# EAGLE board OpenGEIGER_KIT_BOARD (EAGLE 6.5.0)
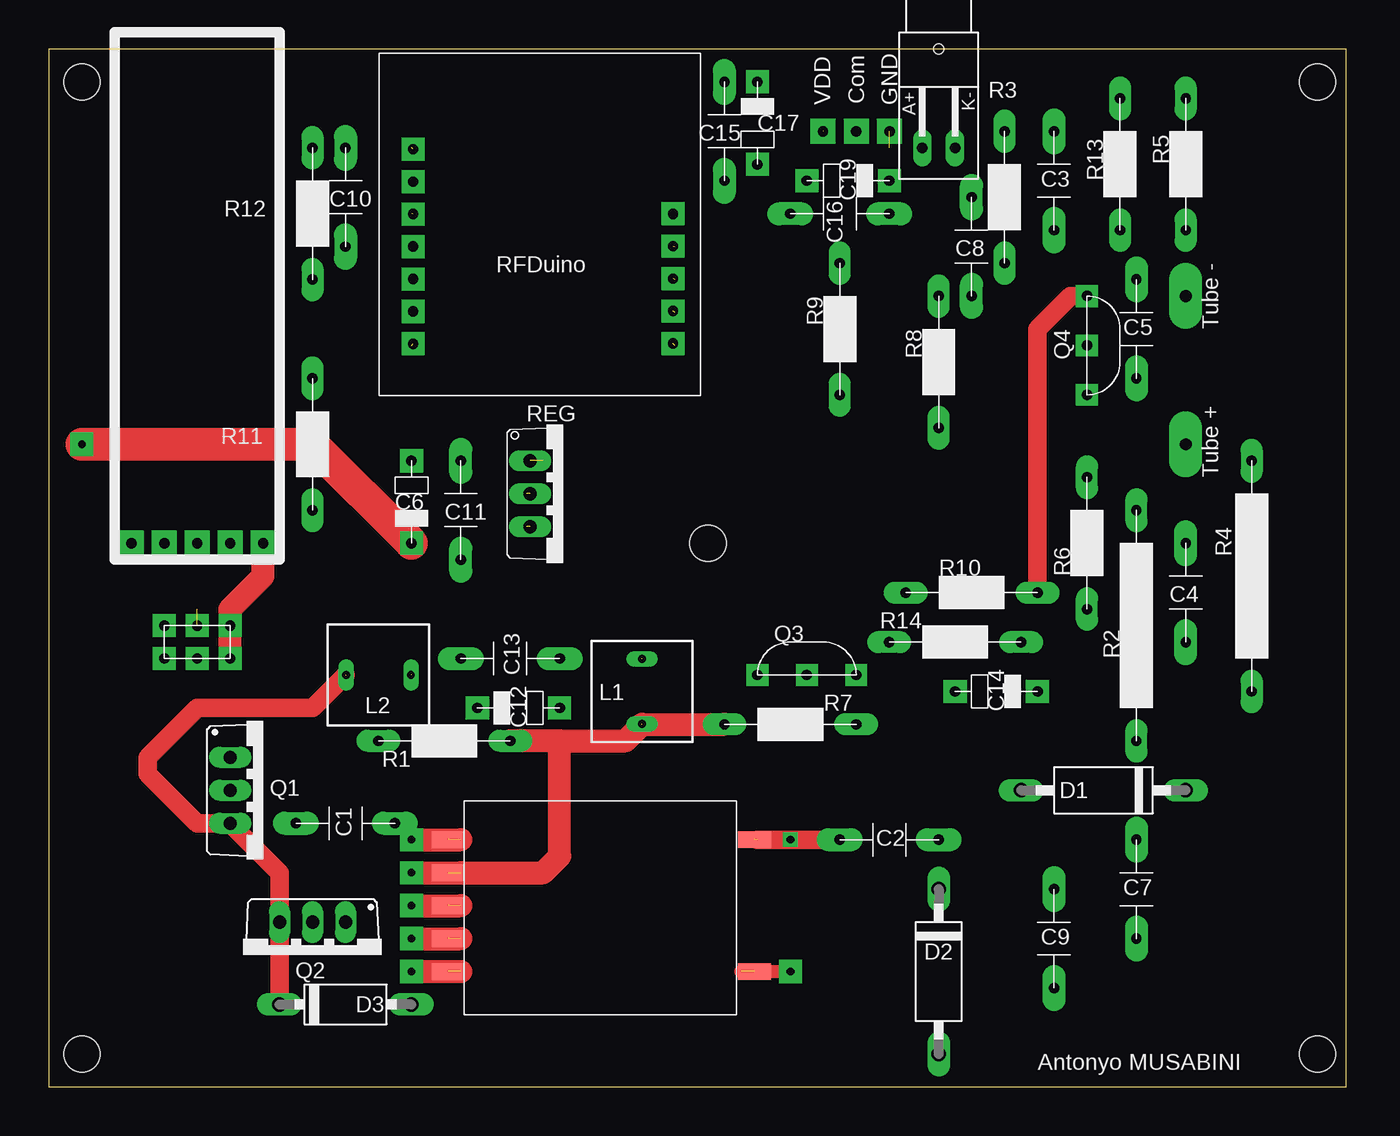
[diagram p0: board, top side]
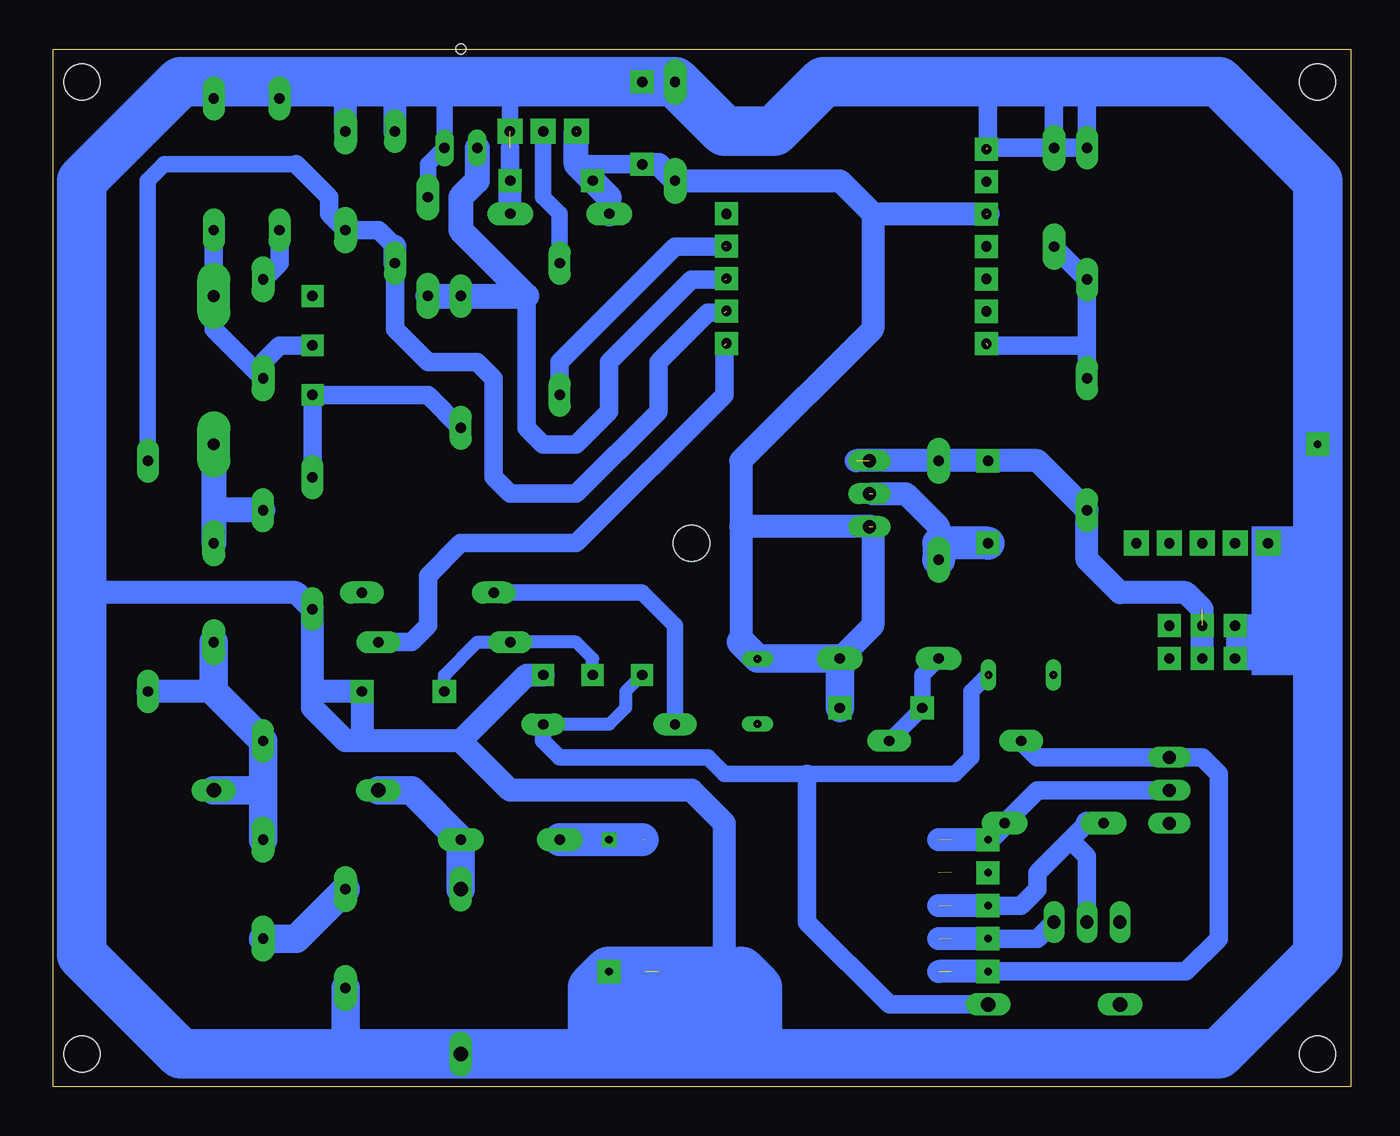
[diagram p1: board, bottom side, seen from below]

Size 100 x 80 mm. Coordinates in mm from the lower left corner, seen from the top.
Outline: 0,0 100,0 100,80 0,80 0,0
Copper layers (1*16): Top 0.035mm / dielectric 1.5mm / Bottom 0.035mm
Design rules "8mils": minimum track width 8mil, minimum drill 20mil, track to track 8mil, track to pad 8mil, pad to pad 8mil, via to via 8mil, smd to smd 8mil, copper to edge 10mil, drill to drill 8mil, minimum pad ring 12mil, minimum via ring 10mil, stop-mask expansion 4mil, vias tented up to drill 25mil, thermal gap 10mil
Holes 2.8 mm at 2.54,77.47 2.54,2.54 97.79,2.54 97.79,77.47 50.8,41.91

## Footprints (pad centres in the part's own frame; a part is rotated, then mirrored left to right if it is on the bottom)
MY_CONDO = drill 0.8 pad 1.778 long: P$1 0,0; P$2 7.62,0
MY_CONDO_CH = drill 0.8 pad 1.778 square: P$1 0,0; P$2 6.35,0
DO15-12 = drill 1.118 long: A 6.35,0; C -6.35,0
P1-10 = drill 1.118 long: A 5.08,0; C -5.08,0
SD8 = drill 0.6 long: 1 -2.5,0; 2 2.5,0
Q62902-B155 = drill 0.813 long: A 7.62,-1.27; K 7.62,1.27 | hole 0.813: 0,0
TO220BV = drill 1.016 long: 1 -2.54,-2.54; 2 0,-2.54; 3 2.54,-2.54
MY_TO92 = drill 0.8 pad 1.676 square: B 3.81,0; C 0,0; E 7.62,0
MY_RESISTANCE = drill 0.8 pad 1.676 long: P$1 0,0; P$2 10.16,0
MY_BIG_R = drill 0.8 pad 1.676 long: P$1 0,0; P$2 17.78,0
TO220V = drill 1.016 long: 1 -2.54,-2.54; 2 0,-2.54; 3 2.54,-2.54
CCFL_TRANSFO = smd 2.54 x 1.27: P$1 -1.238,13.5; P$2 -1.238,10.96; P$3 -1.238,8.42; P$4 -1.238,5.88; P$5 -1.238,3.34; P$6 22.365,3.34; P$10 22.365,13.5
TUBE = drill 0.9 pad 2.54 long: P$1 0,0; P$2 11.43,0
INTERRUPTEUR = drill 0.8 pad 1.778 square: B1 0,-5.08; B2 2.54,-5.08; H1 0,0; H2 2.54,0; M1 0,-2.54; M2 2.54,-2.54
RFDUINO = drill 0.8 pad 1.778 square: +3V 2.606,-12.375; FACTORY 2.606,-17.375; GND 2.606,-7.375; GPIO0/AREF 2.606,-19.875; GPIO1 2.606,-22.375; GPIO2 22.644,-22.35; GPIO3 22.644,-19.85; GPIO4 22.644,-17.35; GPIO5 22.644,-14.85; GPIO6 22.644,-12.35; P2 2.606,-9.875; RESET 2.606,-14.875
CHARGEUR = drill 0.8 pad 1.93 square: P$1 0,0; P$2 0,-2.54; P$3 0,-5.08; P$4 0,-7.62; P$5 0,-10.16
LED_RGB = drill 0.8 pad 1.93 square: COM 0,0; GND 0,2.57; VDD 0,-2.57

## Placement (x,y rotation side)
C1  220n  [MY_CONDO]  19.05,20.32 0 top
C2  47n  [MY_CONDO]  60.96,19.05 0 top
C3  100n  [MY_CONDO]  77.47,73.66 270 top
C4  1n  [MY_CONDO]  87.63,34.29 90 top
C5  10n  [MY_CONDO]  83.82,62.23 270 top
C6  1u  [MY_CONDO_CH]  27.94,48.26 270 top
C7  100n  [MY_CONDO]  83.82,19.05 270 top
C8  100n  [MY_CONDO]  71.12,60.96 90 top
C9  47n  [MY_CONDO]  77.47,15.24 270 top
C10  100n  [MY_CONDO]  22.86,72.39 270 top
C11  100n  [MY_CONDO]  31.75,40.64 90 top
C12  1u  [MY_CONDO_CH]  39.37,29.21 180 top
C13  100n  [MY_CONDO]  31.75,33.02 0 top
C14  1u  [MY_CONDO_CH]  69.85,30.48 0 top
C15  100n  [MY_CONDO]  52.07,77.47 270 top
C16  100n  [MY_CONDO]  64.77,67.31 180 top
C17  1u  [MY_CONDO_CH]  54.61,71.12 90 top
C19  1u  [MY_CONDO_CH]  58.42,69.85 0 top
D1  1N5060GP  [DO15-12]  81.28,22.86 180 top
D2  1N5060GP  [DO15-12]  68.58,8.89 270 top
D3  BA157  [P1-10]  22.86,6.35 0 top
L1  100u  [SD8]  45.72,30.48 90 top
L2  100u  [SD8]  25.4,31.75 180 top
LED1  [Q62902-B155]  68.58,80.01 270 top
Q1  BU505  [TO220BV]  16.51,22.86 270 top
Q2  BU505  [TO220BV]  20.32,10.16 180 top
Q3  BC337  [MY_TO92]  54.61,31.75 0 top
Q4  BC337  [MY_TO92]  80.01,60.96 270 top
R1  330  [MY_RESISTANCE]  25.4,26.67 0 top
R2  4.7M  [MY_BIG_R]  83.82,26.67 90 top
R3  47k  [MY_RESISTANCE]  73.66,73.66 270 top
R4  15M  [MY_BIG_R]  92.71,48.26 270 top
R5  470k  [MY_RESISTANCE]  87.63,76.2 270 top
R6  10k  [MY_RESISTANCE]  80.01,36.83 90 top
R7  1k  [MY_RESISTANCE]  62.23,27.94 180 top
R8  330  [MY_RESISTANCE]  68.58,50.8 90 top
R9  1k  [MY_RESISTANCE]  60.96,53.34 90 top
R10  330  [MY_RESISTANCE]  66.04,38.1 0 top
R11  10k  [MY_RESISTANCE]  20.32,44.45 90 top
R12  33k  [MY_RESISTANCE]  20.32,72.39 270 top
R13  10  [MY_RESISTANCE]  82.55,76.2 270 top
R14  1k  [MY_RESISTANCE]  74.93,34.29 180 top
REG  786TV  [TO220V]  39.62,45.72 270 top
U$1  CCFL_TRANSFO  [CCFL_TRANSFO]  32,5.56 0 top
U$2  TUBE  [TUBE]  87.63,49.53 90 top
U$3  ANTONYO  [ANTONYO]  76.2,1.27 0 top
U$4  INTERRUPTEUR  [INTERRUPTEUR]  13.97,35.56 270 top
U$5  RFDUINO  [RFDUINO]  25.46,79.65 0 top
U$6  CHARGEUR  [CHARGEUR]  6.35,41.91 90 top
U$7  LED_RGB  [LED_RGB]  62.23,73.66 270 top

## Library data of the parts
C1-C17 C19 Q3 Q4 R1-R14 U$1-U$7 = openGeiger
D1-D3 = diode
L1 L2 = inductor-neosid; OC_FARNELL: unknown; OC_NEWARK: unknown
LED1 = led
Q1 Q2 = transistor
REG = linear

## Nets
CHARGEUR+: U$4.H1 U$4.H2 U$6.P$5
COUPS: C8.P$1 LED1.A R8.P$2 U$5.GPIO4
GND: C3.P$1 C6.P$2 C8.P$2 C9.P$2 C10.P$1 C11.P$1 C14.P$2 C15.P$1 C16.P$1 C17.P$2 C19.P$2 D2.A LED1.K Q3.E R3.P$1 R5.P$1 R6.P$1 R12.P$1 R13.P$1 REG.2 U$1.P$6 U$4.B1 U$4.B2 U$5.GND U$6.P$1 U$7.GND
HIGH_V: C4.P$1 C7.P$1 D1.C R2.P$1 R4.P$2
N$1: R9.P$1 U$5.GPIO5
N$2: C7.P$2 C9.P$1
N$3: C2.P$2 D1.A D2.C
N$4: Q1.1 R1.P$1 U$1.P$5
N$5: D3.A L2.1 Q3.C R7.P$1
N$6: C5.P$2 Q4.B R5.P$2 U$2.P$2
N$7: R9.P$2 U$7.COM
N$8: D3.C L2.2 Q1.3 Q2.3
N$9: Q2.1 U$1.P$4
N$10: C10.P$2 R11.P$2 R12.P$2 U$5.GPIO1
N$11: C5.P$1 R13.P$2
N$12: C4.P$2 R2.P$2 U$2.P$1
N$15: Q4.E R6.P$2 R8.P$1
N$17: C1.P$2 Q1.2 U$1.P$1
N$18: C14.P$1 Q3.B R14.P$2
N$19: Q4.C R10.P$2
N$23: C1.P$1 Q2.2 U$1.P$3
N$26: R14.P$1 U$5.GPIO2
N$28: C2.P$1 U$1.P$10
V_SENSE: C3.P$2 R3.P$2 R4.P$1 U$5.GPIO3
VDD_POST_BOBINE: C12.P$2 C13.P$1 L1.1 R1.P$2 R7.P$2 R10.P$1 U$1.P$2
VDD_PRE_REGULATOR: C6.P$1 C11.P$2 R11.P$1 REG.1 U$4.M1 U$4.M2
VDD_PRé_BOBINE: C12.P$1 C13.P$2 C15.P$2 C16.P$2 C17.P$1 C19.P$1 L1.2 REG.3 U$5.+3V U$7.VDD

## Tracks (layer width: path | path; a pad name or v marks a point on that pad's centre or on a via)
CHARGEUR+
  Top 1.778: U$4.H2 U$4.H1 13.97,36.83 16.51,39.37 U$6.P$5
COUPS  (1 unrouted)
  Bottom 1.422: 63.5,60.96 63.5,50.8 62.23,49.53 59.69,49.53 57.15,52.07 57.15,55.88 50.8,62.23 48.26,62.23
  Bottom 1.93: LED1.A 67.31,69.85 68.58,68.58 68.58,66.04 63.5,60.96 R8.P$2 C8.P$1
GND  (via drill 0.6 pad 1.78)  (4 unrouted)
  Top 1.016: 53.34,8.89 v57.15,8.89
  Top 2.54: C6.P$2 20.32,49.53 v2.54,49.53
  Bottom 1.27: R13.P$1 R5.P$1 | C8.P$2 71.12,71.12 LED1.K 69.85,77.47 | 64.77,72.39 64.77,77.47
  Bottom 1.422: C19.P$2 64.77,72.39 | C10.P$1 R12.P$1 20.32,77.47 | C10.P$1 22.86,77.47 | C10.P$1 27.94,72.39 27.94,77.47 | U$4.B2 U$4.B1
  Bottom 1.778: C16.P$1 C19.P$2 | R3.P$1 73.66,77.47 | C3.P$1 77.47,77.47 | R13.P$1 82.55,77.47 | R5.P$1 85.09,77.47 | 77.47,2.54 77.47,3.81 76.2,2.54 D2.A | 46.99,8.89 48.26,8.89 48.26,20.32 50.8,22.86 64.77,22.86 68.58,26.67 | 68.58,26.67 76.2,26.67 | 76.2,26.67 77.47,26.67 80.01,29.21 80.01,30.48 | 80.01,30.48 R6.P$1 81.28,38.1 97.79,38.1 | 68.58,26.67 63.5,31.75 Q3.E | 80.01,30.48 C14.P$2 76.2,26.67 | U$6.P$1 2.54,41.91 | U$4.B1 2.54,35.56 | U$4.B2 2.54,33.02 | 36.83,45.72 34.29,45.72 31.75,43.18 31.75,41.91
  Bottom 2.184: C9.P$2 77.47,3.81
  Bottom 2.54: C11.P$1 31.75,41.91 C6.P$2
  Bottom 3.81: 45.72,2.54 10.16,2.54 2.54,10.16 2.54,33.02 2.54,35.56 2.54,41.91 v2.54,49.53 2.54,69.85 10.16,77.47 20.32,77.47 22.86,77.47 27.94,77.47 40.64,77.47 44.45,73.66 48.26,73.66 C15.P$1 C17.P$2 64.77,77.47 69.85,77.47 73.66,77.47 77.47,77.47 82.55,77.47 85.09,77.47 90.17,77.47 97.79,69.85 97.79,38.1 97.79,10.16 90.17,2.54 77.47,2.54 D2.A 58.42,2.54 | 45.72,2.54 58.42,2.54 | 58.42,2.54 58.42,7.62 v57.15,8.89 48.26,8.89 | 46.99,8.89 45.72,7.62 45.72,2.54
HIGH_V
  Bottom 1.778: 87.63,30.48 R4.P$2
  Bottom 2.184: C4.P$1 87.63,30.48 R2.P$1 83.82,22.86 | 83.82,22.86 C7.P$1 | 83.82,22.86 D1.C
N$1  (1 unrouted)
  Bottom 1.422: R9.P$1 60.96,55.88 52.07,64.77 48.26,64.77
N$2
  Bottom 2.184: C9.P$1 81.28,11.43 C7.P$2
N$3
  Bottom 2.184: D2.C C2.P$2 72.39,22.86 D1.A
N$4  (via drill 0.6 pad 1.78)  (1 unrouted)
  Top 1.778: v27.94,8.89 31.75,8.89
  Bottom 1.422: R1.P$1 24.13,25.4 Q1.1 11.43,25.4 10.16,24.13 10.16,11.43 12.7,8.89 v27.94,8.89
  Bottom 1.778: v27.94,8.89 31.75,8.89
N$5  (1 unrouted)
  Bottom 1.016: Q3.C 55.88,30.48 55.88,29.21 57.15,27.94 R7.P$1
  Bottom 1.27: 27.94,31.75 29.21,30.48 29.21,25.4 30.48,24.13 41.91,24.13 48.26,24.13 49.53,25.4 60.96,25.4 62.23,26.67 R7.P$1
  Bottom 1.422: D3.A 35.56,6.35 41.91,12.7 41.91,24.13
N$6
  Bottom 1.422: R5.P$2 U$2.P$2 87.63,58.42 C5.P$2 83.82,55.88 82.55,57.15 Q4.B
  Bottom 1.93: 87.63,59.69 U$2.P$2
N$7
  Bottom 1.27: R9.P$2 60.96,67.31 62.23,68.58 U$7.COM
N$8  (1 unrouted)
  Top 1.422: D3.C Q2.3 17.78,16.51 Q1.3 11.43,20.32 7.62,24.13 7.62,25.4 11.43,29.21 20.32,29.21 22.86,31.75
N$9  (via drill 0.6 pad 1.78)  (1 unrouted)
  Top 1.778: v27.94,11.43 31.75,11.43
  Bottom 1.422: Q2.1 24.13,11.43 v27.94,11.43
  Bottom 1.778: v27.94,11.43 31.75,11.43
N$10  (1 unrouted)
  Bottom 1.422: C10.P$2 R12.P$2 20.32,57.15 | R11.P$2 20.32,57.15 | 27.94,57.15 20.32,57.15
N$11
  Bottom 1.422: R13.P$2 82.55,63.5 C5.P$1
N$12
  Bottom 1.93: R2.P$2 87.63,44.45 | U$2.P$1 87.63,44.45 | 87.63,44.45 C4.P$2
N$15
  Bottom 1.422: R8.P$1 71.12,53.34 Q4.E R6.P$2
N$17  (via drill 0.6 pad 1.78)  (1 unrouted)
  Top 1.778: v27.94,19.05 31.75,19.05
  Bottom 1.422: Q1.2 24.13,22.86 C1.P$2
  Bottom 1.778: C1.P$2 v27.94,19.05 31.75,19.05
N$18
  Bottom 1.016: Q3.B 58.42,33.02 59.69,34.29 63.5,34.29 R14.P$2 67.31,34.29 69.85,31.75 C14.P$1
N$19
  Top 1.422: Q4.C 78.74,60.96 76.2,58.42 R10.P$2
N$23  (via drill 0.6 pad 1.78)  (1 unrouted)
  Top 1.778: v27.94,13.97 31.75,13.97
  Bottom 1.422: 20.32,13.97 Q2.2 20.32,17.78 21.59,19.05 | 20.32,20.32 21.59,19.05 | 21.59,19.05 24.13,16.51 24.13,15.24 25.4,13.97 v27.94,13.97
  Bottom 1.778: C1.P$1 20.32,20.32 | v27.94,13.97 31.75,13.97
N$26  (1 unrouted)
  Bottom 1.422: 48.26,57.15 48.26,53.34 59.69,41.91 68.58,41.91 71.12,39.37 71.12,35.56 72.39,34.29 R14.P$1
N$28  (via drill 0.6)  (1 unrouted)
  Top 1.422: 54.61,19.05 v57.15,19.05 C2.P$1
  Bottom 2.54: 54.61,19.05 v57.15,19.05 C2.P$1
V_SENSE  (1 unrouted)
  Bottom 1.27: 81.28,71.12 91.44,71.12 92.71,69.85 R4.P$1
  Bottom 1.422: R3.P$2 73.66,58.42 71.12,55.88 67.31,55.88 66.04,54.61 66.04,46.99 64.77,45.72 59.69,45.72 53.34,52.07 53.34,55.88 49.53,59.69 48.26,59.69 | 73.66,64.77 74.93,66.04 C3.P$2 78.74,67.31 78.74,68.58 81.28,71.12
  Bottom 1.778: R3.P$2 73.66,64.77
VDD_POST_BOBINE  (via drill 0.6 pad 1.78)  (2 unrouted)
  Top 1.778: 31.75,16.51 v27.94,16.51 38.1,16.51 39.37,17.78 39.37,26.67 | 39.37,26.67 44.45,26.67 45.72,27.94 R7.P$2 | 39.37,26.67 R1.P$2
  Bottom 1.27: C13.P$1 33.02,31.75 C12.P$2 R1.P$2 | R7.P$2 52.07,35.56 54.61,38.1 R10.P$1
VDD_PRE_REGULATOR  (2 unrouted)
  Bottom 1.778: U$4.M2 11.43,36.83 12.7,38.1 17.78,38.1 20.32,40.64 R11.P$1 24.13,48.26 C6.P$1 C11.P$2 38.1,48.26
VDD_PRé_BOBINE  (4 unrouted)
  Bottom 1.422: C17.P$1 59.69,71.12
  Bottom 1.778: C17.P$1 53.34,71.12 C15.P$2 39.37,69.85 36.83,67.31 | 36.83,67.31 27.94,67.31 | 36.83,67.31 36.83,58.42 46.99,48.26 46.99,43.18 | 46.99,43.18 46.99,34.29 | 46.99,43.18 36.83,43.18 36.83,35.56 C13.P$2
  Bottom 1.93: C16.P$2 57.15,68.58 C19.P$1 59.69,71.12 59.69,73.66
  Bottom 2.184: C12.P$1 C13.P$2 45.72,33.02 46.99,34.29
(copper drawn outside any net)
  shapes: Bottom area x3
